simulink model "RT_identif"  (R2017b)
settings: Solver=ode1  StartTime=0.0  StopTime=30  FixedStep=0.001  RelTol=1e-3
undefined symbols (not defined in the file or in its folder): Advantech, PCI
libraries: sldrtlib x11

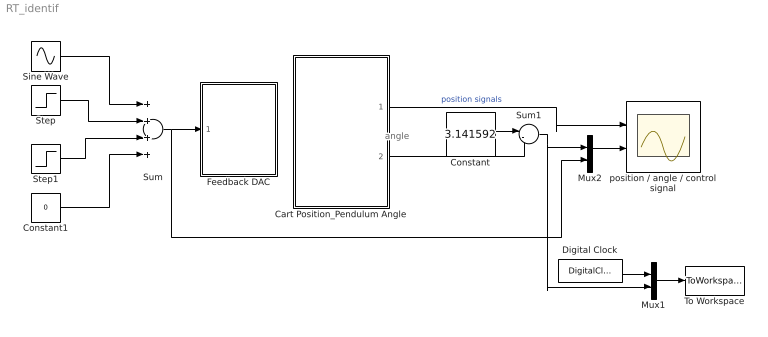
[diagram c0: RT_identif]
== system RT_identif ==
  note: angle
  Cart Position_Pendulum Angle : Subsystem  mask(Feedback Encoder Block){st=0.001, of1=0, of2=-1024}
      mask prompts: st "Sample Time"; of1 "Channel 1 Offset"; of2 "Channel 2 Offset"
      mask help: Special block to use with the Feedback experiments to read encoder channels using the digital I/O lines
  Constant : Constant  Value=3.141592
  Constant1 : Constant  Value=0
  Digital Clock : DigitalClock  SampleTime=0.001
  Feedback DAC : Subsystem  mask(DAC Unit for Feedback Experiments){st=0.001, ch=1}
      mask prompts: st "Sample Time"; ch "Output Channel"
      mask help: Digital to Analog Output for Feedback Experiments using Advantech PCI1711 I/O board
  Mux1 : Mux  Inputs=2
  Mux2 : Mux  Inputs=2
  Sine Wave : Sin  Amplitude=0  Frequency=5  SampleTime=0
  Step : Step  Time=5  After=0  SampleTime=0
  Step1 : Step  Time=2  After=0  SampleTime=0
  Sum : Sum  Inputs=++++
  Sum1 : Sum  Inputs=|-+
  To Workspace : ToWorkspace  VariableName=teta_mes  SampleTime=-1
  position / angle / control signal : Scope  NumInputPorts=2
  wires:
  Mux2/1 -> position / angle / control signal/2
  Step1/1 -> Sum/3
  Step/1 -> Sum/2
  Sine Wave/1 -> Sum/1
  Constant/1 -> Sum1/1
  Cart Position_Pendulum Angle/2(Channel 2) -> Sum1/2
  Sum1/1 -> Mux1/2, Mux2/1
  Sum/1 -> Mux2/2, Feedback DAC/1(In1)
  Constant1/1 -> Sum/4
  Mux1/1 -> To Workspace/1
  Digital Clock/1 -> Mux1/1
  Cart Position_Pendulum Angle/1(Channel 1) -> position / angle / control signal/1  "position signals"

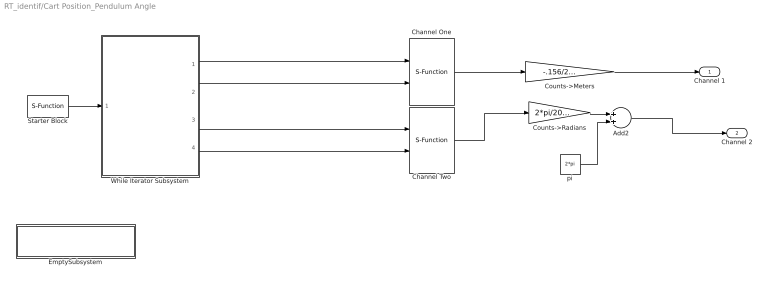
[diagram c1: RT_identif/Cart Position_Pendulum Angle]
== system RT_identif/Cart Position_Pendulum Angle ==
  Add2 : Sum
  Channel One : S-Function  FunctionName=Converter  Parameters=of1,st  SFunctionDeploymentMode=off  EnableBusSupport=off
  Channel Two : S-Function  FunctionName=Converter  Parameters=of2,st  SFunctionDeploymentMode=off  EnableBusSupport=off
  Counts->Meters : Gain  Gain=-.156/2048
  Counts->Radians : Gain  Gain=2*pi/2048
  EmptySubsystem : Subsystem
  Starter Block : S-Function  FunctionName=Starter  Parameters=sample_time  SFunctionDeploymentMode=off  EnableBusSupport=off  mask{sample_time=st}
      mask prompts: sample_time "Sample Time:"
  While Iterator Subsystem : Subsystem  TreatAsAtomicUnit=on
  pi : Constant  Value=2*pi
  Channel 1 : Outport
  Channel 2 : Outport  Port=2
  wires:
  Add2/1 -> Channel 2/1
  Channel Two/1 -> Counts->Radians/1
  pi/1 -> Add2/2
  Counts->Radians/1 -> Add2/1
  Counts->Meters/1 -> Channel 1/1
  Starter Block/1 -> While Iterator Subsystem/1(In1)
  While Iterator Subsystem/1(Out1) -> Channel One/1
  While Iterator Subsystem/2(Out3) -> Channel One/2
  While Iterator Subsystem/3(Out2) -> Channel Two/1
  While Iterator Subsystem/4(Out4) -> Channel Two/2
  Channel One/1 -> Counts->Meters/1

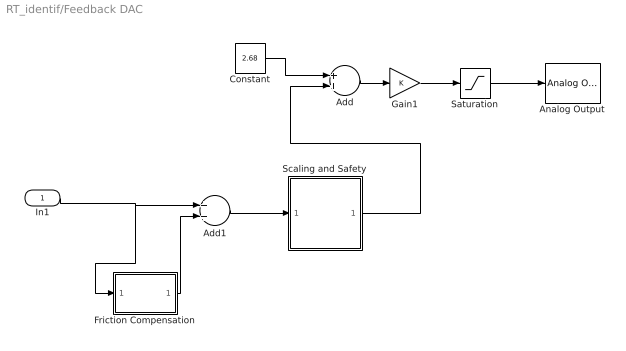
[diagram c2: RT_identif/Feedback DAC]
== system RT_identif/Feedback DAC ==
  In1 : Inport
  Add : Sum
  Add1 : Sum
  Analog Output : sldrtlib/Analog Output  SampleTime=st  MaxMissedTicks=10  ShowMissedTicks=off  YieldWhenWaiting=off  DrvName=Advantech/PCI-1711  DrvAddress=4294967295  DrvOptions=zeros(1,0)  Channels=ch  RangeMode=1  VoltRange=2  InitialValue=2.5  FinalValue=2.5
  Constant : Constant  Value=2.68
  Friction Compensation : Subsystem  mask(linear){frictionCompNeg=.1, frictionCompPos=.1}
      mask prompts: frictionCompNeg "Friction Compensation Magnitude in Negative Direction"; frictionCompPos "Friction Compensation Magnitude in Positive Direction"
  Gain1 : Gain
  Saturation : Saturate  UpperLimit=5.0  LowerLimit=0
  Scaling and Safety : Subsystem
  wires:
  Scaling and Safety/1(Out1) -> Add/2
  Gain1/1 -> Saturation/1
  Add/1 -> Gain1/1
  Saturation/1 -> Analog Output/1
  Constant/1 -> Add/1
  Friction Compensation/1(Out1) -> Add1/2
  In1/1 -> Friction Compensation/1(In1), Add1/1
  Add1/1 -> Scaling and Safety/1(In1)

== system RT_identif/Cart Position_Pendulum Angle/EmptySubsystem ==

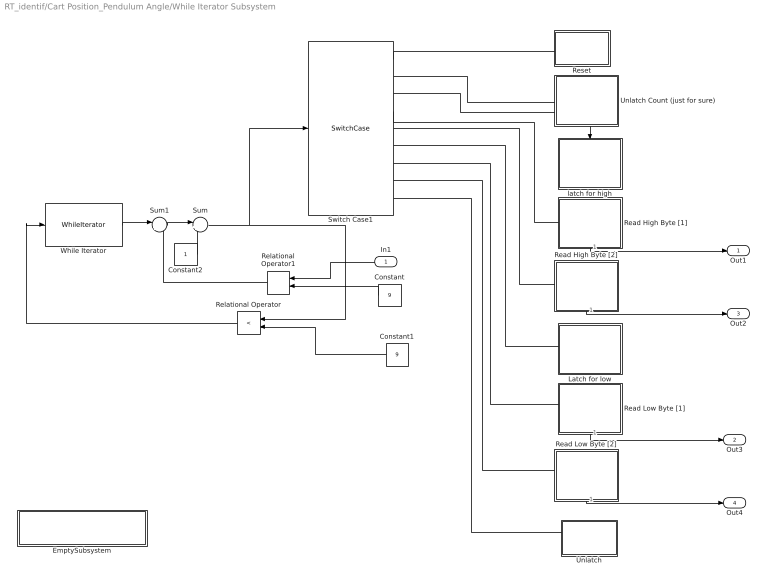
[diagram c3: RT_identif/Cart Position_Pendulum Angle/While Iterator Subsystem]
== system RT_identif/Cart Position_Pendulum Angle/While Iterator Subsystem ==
  In1 : Inport
  Constant : Constant  Value=9
  Constant1 : Constant  Value=9
  Constant2 : Constant
  EmptySubsystem : Subsystem
  Latch for low : Subsystem  TreatAsAtomicUnit=on
  Read High Byte [1] : Subsystem  TreatAsAtomicUnit=on
  Read High Byte [2] : Subsystem  TreatAsAtomicUnit=on
  Read Low Byte [1] : Subsystem  TreatAsAtomicUnit=on
  Read Low Byte [2] : Subsystem  TreatAsAtomicUnit=on
  Relational Operator : RelationalOperator  Operator=<  OutDataTypeStr=boolean
  Relational Operator1 : RelationalOperator  Operator===  OutDataTypeStr=boolean
  Reset : Subsystem  TreatAsAtomicUnit=on
  Sum : Sum  Inputs=|++
  Sum1 : Sum  Inputs=|+-
  Switch Case1 : SwitchCase  CaseConditions={1,2,3,4,5,6,7,8,9}  ShowDefaultCase=off
  Unlatch : Subsystem  TreatAsAtomicUnit=on
  "Unlatch Count (just for sure) " : Subsystem  TreatAsAtomicUnit=on
  While Iterator : WhileIterator  MaxIters=9  WhileBlockType=do-while  ResetStates=reset  ShowIterationPort=on  OutputDataType=int8
  latch for high : Subsystem  TreatAsAtomicUnit=on
  Out1 : Outport
  Out3 : Outport  Port=2
  Out2 : Outport  Port=3
  Out4 : Outport  Port=4
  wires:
  Relational Operator/1 -> While Iterator/1
  In1/1 -> Relational Operator1/1
  Constant/1 -> Relational Operator1/2
  Relational Operator1/1 -> Sum1/2
  While Iterator/1 -> Sum1/1
  Switch Case1/1 -> Reset/Action
  Switch Case1/2 -> "Unlatch Count (just for sure) "/Action
  Constant1/1 -> Relational Operator/2
  Read High Byte [1]/1(Out2) -> Out1/1
  Read High Byte [2]/1(Out2) -> Out2/1
  Read Low Byte [1]/1(Out2) -> Out3/1
  Read Low Byte [2]/1(Out2) -> Out4/1
  Sum1/1 -> Sum/1
  Sum/1 -> Switch Case1/1, Relational Operator/1
  Constant2/1 -> Sum/2
  Switch Case1/3 -> latch for high/Action
  Switch Case1/4 -> Read High Byte [1]/Action
  Switch Case1/5 -> Read High Byte [2]/Action
  Switch Case1/6 -> Latch for low/Action
  Switch Case1/7 -> Read Low Byte [1]/Action
  Switch Case1/8 -> Read Low Byte [2]/Action
  Switch Case1/9 -> Unlatch/Action

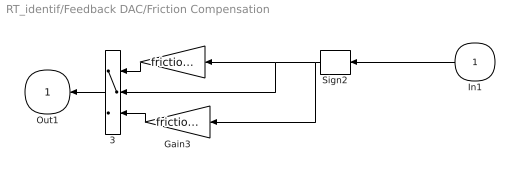
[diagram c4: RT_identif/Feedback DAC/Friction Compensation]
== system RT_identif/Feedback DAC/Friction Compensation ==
  In1 : Inport
  " " : Gain  Gain=frictionCompPos
  3 : Switch
  Gain3 : Gain  Gain=frictionCompNeg
  Sign2 : Signum  Tag=T
  Out1 : Outport  InitialOutput=0
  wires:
  In1/1 -> Sign2/1
  " "/1 -> 3/1
  Gain3/1 -> 3/3
  Sign2/1 -> Gain3/1, " "/1, 3/2
  3/1 -> Out1/1

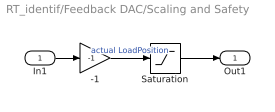
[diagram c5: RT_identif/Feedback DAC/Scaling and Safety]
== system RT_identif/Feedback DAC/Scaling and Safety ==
  In1 : Inport
  -1 : Gain  Gain=-1
  Saturation : Saturate  UpperLimit=2.5  LowerLimit=-2.5
  Out1 : Outport
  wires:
  Saturation/1 -> Out1/1
  In1/1 -> -1/1
  -1/1 -> Saturation/1  "actual LoadPosition"

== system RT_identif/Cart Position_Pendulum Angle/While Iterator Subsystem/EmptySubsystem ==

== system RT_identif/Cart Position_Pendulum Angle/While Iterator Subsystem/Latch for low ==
  Action Port : ActionPort  ActionType=case
  Constant : Constant  Value=6  OutDataTypeStr=double
  Digital Output : sldrtlib/Digital Output  SampleTime=-1  MaxMissedTicks=10  ShowMissedTicks=off  YieldWhenWaiting=off  DrvName=Advantech/PCI-1711  DrvAddress=4294967295  DrvOptions=zeros(1,0)  Channels=1  BitMode=2  InitialValue=0  FinalValue=0
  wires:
  Constant/1 -> Digital Output/1

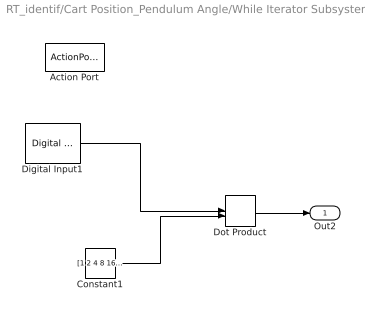
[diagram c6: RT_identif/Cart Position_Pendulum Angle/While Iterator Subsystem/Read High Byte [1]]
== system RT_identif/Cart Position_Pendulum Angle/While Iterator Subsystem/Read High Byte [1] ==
  Action Port : ActionPort  ActionType=case
  Constant1 : Constant  Value=[1 2 4 8 16 32 64 128]
  Digital Input1 : sldrtlib/Digital Input  SampleTime=-1  MaxMissedTicks=10  ShowMissedTicks=off  YieldWhenWaiting=off  DrvName=Advantech/PCI-1711  DrvAddress=4294967295  DrvOptions=zeros(1,0)  Channels=[1,2,3,4,5,6,7,8]  BitMode=1  DataType=1
  Dot Product : DotProduct
  Out2 : Outport
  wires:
  Dot Product/1 -> Out2/1
  Constant1/1 -> Dot Product/2
  Digital Input1/1 -> Dot Product/1

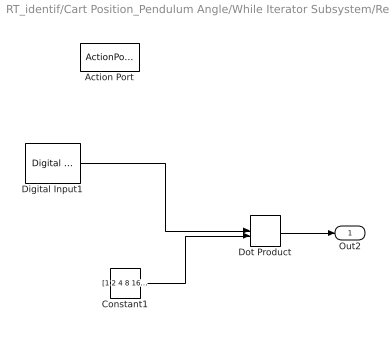
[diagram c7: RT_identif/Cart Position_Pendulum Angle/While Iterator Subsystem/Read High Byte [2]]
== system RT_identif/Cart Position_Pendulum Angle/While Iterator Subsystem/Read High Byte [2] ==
  Action Port : ActionPort  ActionType=case
  Constant1 : Constant  Value=[1 2 4 8 16 32 64 128]
  Digital Input1 : sldrtlib/Digital Input  SampleTime=-1  MaxMissedTicks=10  ShowMissedTicks=off  YieldWhenWaiting=off  DrvName=Advantech/PCI-1711  DrvAddress=4294967295  DrvOptions=zeros(1,0)  Channels=[9:16]  BitMode=1  DataType=1
  Dot Product : DotProduct
  Out2 : Outport
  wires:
  Digital Input1/1 -> Dot Product/1
  Constant1/1 -> Dot Product/2
  Dot Product/1 -> Out2/1

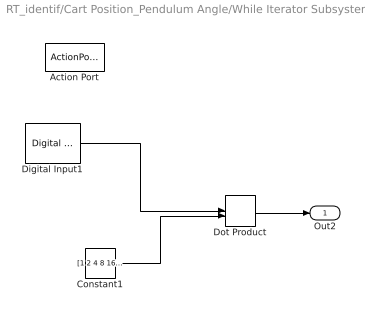
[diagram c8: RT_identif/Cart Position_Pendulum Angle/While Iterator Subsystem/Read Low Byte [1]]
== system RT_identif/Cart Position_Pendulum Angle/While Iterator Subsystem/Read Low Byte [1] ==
  Action Port : ActionPort  ActionType=case
  Constant1 : Constant  Value=[1 2 4 8 16 32 64 128]
  Digital Input1 : sldrtlib/Digital Input  SampleTime=-1  MaxMissedTicks=10  ShowMissedTicks=off  YieldWhenWaiting=off  DrvName=Advantech/PCI-1711  DrvAddress=4294967295  DrvOptions=zeros(1,0)  Channels=[1:8]  BitMode=1  DataType=1
  Dot Product : DotProduct
  Out2 : Outport
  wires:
  Digital Input1/1 -> Dot Product/1
  Constant1/1 -> Dot Product/2
  Dot Product/1 -> Out2/1

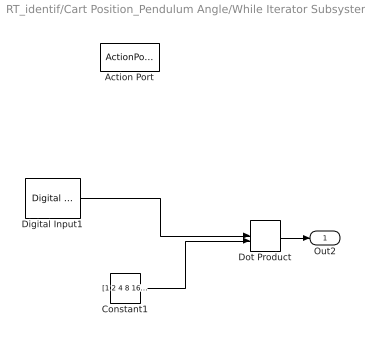
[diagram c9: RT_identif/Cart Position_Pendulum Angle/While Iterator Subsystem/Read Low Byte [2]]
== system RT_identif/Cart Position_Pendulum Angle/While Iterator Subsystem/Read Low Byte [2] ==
  Action Port : ActionPort  ActionType=case
  Constant1 : Constant  Value=[1 2 4 8 16 32 64 128]
  Digital Input1 : sldrtlib/Digital Input  SampleTime=-1  MaxMissedTicks=10  ShowMissedTicks=off  YieldWhenWaiting=off  DrvName=Advantech/PCI-1711  DrvAddress=4294967295  DrvOptions=zeros(1,0)  Channels=[9:16]  BitMode=1  DataType=1
  Dot Product : DotProduct
  Out2 : Outport
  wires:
  Constant1/1 -> Dot Product/2
  Digital Input1/1 -> Dot Product/1
  Dot Product/1 -> Out2/1

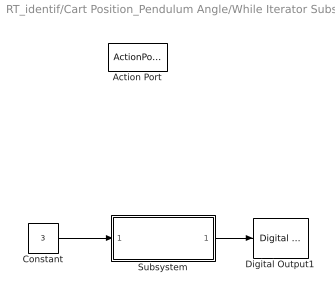
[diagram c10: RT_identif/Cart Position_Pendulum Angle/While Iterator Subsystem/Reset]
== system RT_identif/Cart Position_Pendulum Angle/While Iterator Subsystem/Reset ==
  Action Port : ActionPort  ActionType=case
  Constant : Constant  Value=3  OutDataTypeStr=double
  Digital Output1 : sldrtlib/Digital Output  SampleTime=-1  MaxMissedTicks=10  ShowMissedTicks=off  YieldWhenWaiting=off  DrvName=Advantech/PCI-1711  DrvAddress=4294967295  DrvOptions=zeros(1,0)  Channels=1  BitMode=2  InitialValue=0  FinalValue=0
  Subsystem : Subsystem
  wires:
  Constant/1 -> Subsystem/1(In1)
  Subsystem/1(Out1) -> Digital Output1/1

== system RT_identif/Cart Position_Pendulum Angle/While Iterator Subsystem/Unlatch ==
  Action Port : ActionPort  ActionType=case
  Constant : Constant  Value=7  OutDataTypeStr=double
  Digital Output1 : sldrtlib/Digital Output  SampleTime=-1  MaxMissedTicks=10  ShowMissedTicks=off  YieldWhenWaiting=off  DrvName=Advantech/PCI-1711  DrvAddress=4294967295  DrvOptions=zeros(1,0)  Channels=1  BitMode=2  InitialValue=0  FinalValue=0
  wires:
  Constant/1 -> Digital Output1/1

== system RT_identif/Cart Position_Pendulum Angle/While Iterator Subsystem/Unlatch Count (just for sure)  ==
  Action Port : ActionPort  ActionType=case
  Constant : Constant  Value=7  OutDataTypeStr=double
  Digital Output : sldrtlib/Digital Output  SampleTime=-1  MaxMissedTicks=10  ShowMissedTicks=off  YieldWhenWaiting=off  DrvName=Advantech/PCI-1711  DrvAddress=4294967295  DrvOptions=zeros(1,0)  Channels=1  BitMode=2  InitialValue=0  FinalValue=0
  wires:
  Constant/1 -> Digital Output/1

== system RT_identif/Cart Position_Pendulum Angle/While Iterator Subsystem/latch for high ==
  Action Port : ActionPort  ActionType=case
  Constant : Constant  Value=4  OutDataTypeStr=double
  Digital Output : sldrtlib/Digital Output  SampleTime=-1  MaxMissedTicks=10  ShowMissedTicks=off  YieldWhenWaiting=off  DrvName=Advantech/PCI-1711  DrvAddress=4294967295  DrvOptions=zeros(1,0)  Channels=1  BitMode=2  InitialValue=0  FinalValue=0
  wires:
  Constant/1 -> Digital Output/1

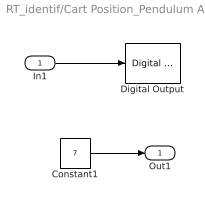
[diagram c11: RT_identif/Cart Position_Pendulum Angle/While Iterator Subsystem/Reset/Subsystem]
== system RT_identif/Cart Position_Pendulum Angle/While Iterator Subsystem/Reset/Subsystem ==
  In1 : Inport
  Constant1 : Constant  Value=7  OutDataTypeStr=double
  Digital Output : sldrtlib/Digital Output  SampleTime=-1  MaxMissedTicks=10  ShowMissedTicks=off  YieldWhenWaiting=off  DrvName=Advantech/PCI-1711  DrvAddress=4294967295  DrvOptions=zeros(1,0)  Channels=[1 2 3]  BitMode=2  InitialValue=0  FinalValue=0
  Out1 : Outport
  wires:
  Constant1/1 -> Out1/1
  In1/1 -> Digital Output/1
